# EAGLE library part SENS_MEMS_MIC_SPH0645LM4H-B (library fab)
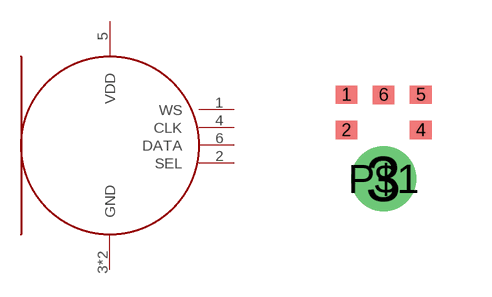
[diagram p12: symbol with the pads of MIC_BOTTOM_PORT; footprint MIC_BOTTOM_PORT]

Designator prefix -

## SENS_MEMS_MIC_SPH0645LM4H-BI2S  [MIC_BOTTOM_PORT]
1  WS
2  SEL
3  GND
4  CLK
5  VDD
6  DATA
P$1  GND

## Footprint MIC_BOTTOM_PORT (pad centres in mm)
Knowles SPH0645LM4H-B I2S Output Digital Microphone, 18-bit precision
smd 0.54 x 0.46: 1 -0.929,2.106; 2 -0.931,1.221; 4 0.931,1.22; 5 0.93,2.105; 6 0,2.102
smd 1.624 x 1.624: 3 0,0
drill 1.024 pad 1.624: P$1 0,0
